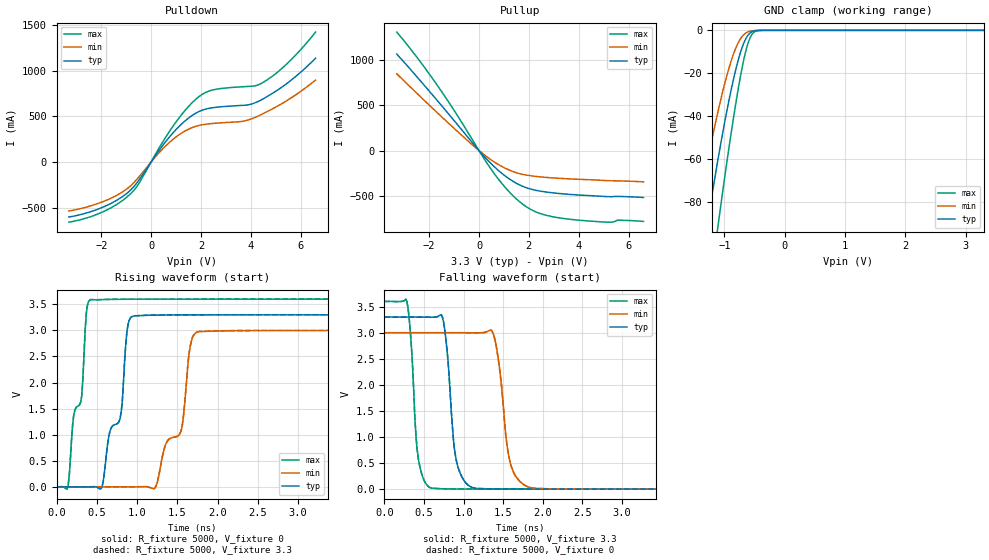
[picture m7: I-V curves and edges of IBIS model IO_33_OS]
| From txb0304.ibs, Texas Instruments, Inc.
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[Model]   IO_33_OS
Model_type  I/O
Vinl=1.05
Vinh=2.34
Enable   Active-High
Vref =   0
Rref =   5000
Cref =   15p
Vmeas =   1.65
| variable   typ   min   max
C_comp   3.56pF   3.29pF   3.85pF
| C_pullup   6.78pF   4.93pF   8.55pF
| C_pulldown   6.52pF   2.81pF   9.96pF
| C_tri-state   3.56pF   3.29pF   3.85pF
[Temperature Range]   40   100   -40
| Ambient temperature   25   85   -40
[Voltage range]   3.3   3   3.6
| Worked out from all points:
|   slope of the pulldown table from 0 to 0.495 V, typ, clamps not added: 2.58 ohm
|   slope of the pullup table from 0 to 0.495 V, typ, clamps not added: 3.39 ohm
|   GND clamp passes 1 mA (typ) near -0.56 V on its own axis
|   rising waveform, R_fixture 5000, V_fixture 0: 20-80 % time 234ps typ, 317ps min, 172ps max; typ from 0 V to 3.3 V
|   falling waveform, R_fixture 5000, V_fixture 3.3: 20-80 % time 103ps typ, 128ps min, 82.7ps max; typ from 3.3 V to 0.002 V
|   rising waveform, R_fixture 5000, V_fixture 3.3: 20-80 % time 234ps typ, 317ps min, 172ps max; typ from 0.002 V to 3.3 V
|   falling waveform, R_fixture 5000, V_fixture 0: 20-80 % time 103ps typ, 128ps min, 82.7ps max; typ from 3.3 V to 0 V
[GND Clamp]
| IO_33
|   Voltage   I(typ)   I(min)   I(max)
-3.3V     -511mA     -429.4mA   -605.2mA
-1.49V    -128.8mA   -92.59mA   -176mA
-1.305V   -94.44mA   -64.67mA   -134.3mA
-1.27V    -88.18mA   -59.68mA   -126.6mA
-1.105V   -60.01mA   -37.73mA   -91.07mA
-955mV    -36.96mA   -20.66mA   -60.66mA
-835mV    -21.06mA   -9.955mA   -38.29mA
-710mV    -8.29mA    -2.997mA   -17.96mA
-620mV    -2.726mA   -874.7uA   -7.07mA
-530mV    -508.5uA   -191.3uA   -1.442mA
-410mV    -26.79uA   -12.71uA   -53.57uA
3.3V      1.563nA    31.42nA    89.95pA
[Pulldown]
| IO_33
|   Voltage   I(typ)   I(min)   I(max)
-3.3V     -601.6mA   -536.2mA   -657.8mA
-1.9V     -489.5mA   -429.7mA   -540.3mA
-815mV    -303.8mA   -258.4mA   -344.5mA
-505mV    -203.4mA   -167.4mA   -240mA
755mV     280mA      219.3mA    342.4mA
1.365V    450.2mA    339.9mA    565.3mA
1.915V    551.4mA    399.5mA    713.7mA
2.525V    595.7mA    423.1mA    791.4mA
3.695V    620.1mA    446.7mA    823.6mA
4.46V     685.1mA    525mA      865.1mA
5.455V    860.5mA    672.7mA    1.075A
6.6V      1.135A     896.9mA    1.421A
[Pullup]
| IO_33
|   Voltage   I(typ)   I(min)   I(max)
-3.3V     1.06A      843.1mA    1.301A
-2.485V   808.2mA    627.1mA    1.022A
-1.625V   533.5mA    403.2mA    697.3mA
-850mV    280.2mA    206.8mA    377.5mA
120mV     -37.65mA   -26.89mA   -53.09mA
950mV     -257.4mA   -179.2mA   -371.9mA
1.73V     -389.7mA   -260mA     -583.6mA
2.385V    -441.5mA   -286.7mA   -684.7mA
3.28V     -472.9mA   -305.6mA   -741.3mA
5.115V    -505mA     -329.5mA   -785.6mA
5.595V    -503.5mA   -332.8mA   -764.8mA
6.6V      -515.1mA   -343.1mA   -777.6mA
[Ramp]
| IO_33
| variable   typ   min   max
dV/dt_r   2.00/2.37E-10   1.82/3.20E-10   2.19/1.73E-10
dV/dt_f   2.01/1.08E-10   1.83/1.34E-10   2.19/8.63E-11
R_load = 5000
[Rising Waveform]
| IO_33
R_fixture =   5000
C_fixture =   0
L_fixture =   0
V_fixture =   0
V_fixture_min = 0
V_fixture_max = 0
|   Time   V(typ)   V(min)   V(max)
0s        1.658nV    7.82nV     214.9pV
145ps     -6.519uV   48.58nV    31.42mV
425ps     1.627mV    -563.8nV   3.59V
789ps     1.307V     13.49uV    3.595V
901ps     3.187V     -93.83uV   3.596V
1.139ns   3.289V     -3.05mV    3.597V
1.545ns   3.296V     1.064V     3.598V
1.699ns   3.297V     2.9V       3.598V
1.993ns   3.297V     2.988V     3.598V
67.55ns   3.298V     2.997V     3.598V
[Falling Waveform]
| IO_33
R_fixture =   5000
C_fixture =   0
L_fixture =   0
V_fixture =   3.3
V_fixture_min = 3
V_fixture_max = 3.6
|   Time   V(typ)   V(min)   V(max)
0s        3.3V       3V         3.6V
285ps     3.3V       3V         3.59V
439ps     3.3V       3V         487mV
719ps     3.345V     3V         8.876mV
915ps     500.4mV    3V         3.753mV
1.265ns   9.382mV    3.006V     2.028mV
1.405ns   5.05mV     2.794V     1.824mV
1.601ns   2.935mV    436mV      1.666mV
1.937ns   1.992mV    13.15mV    1.545mV
67.55ns   1.582mV    1.775mV    1.448mV
[Rising Waveform]
| IO_33
R_fixture =   5000
C_fixture =   0
L_fixture =   0
V_fixture =   3.3
V_fixture_min = 3
V_fixture_max = 3.6
|   Time   V(typ)   V(min)   V(max)
0s        1.582mV    1.775mV    1.448mV
145ps     1.576mV    1.775mV    32.87mV
425ps     3.21mV     1.774mV    3.591V
789ps     1.309V     1.788mV    3.597V
901ps     3.19V      1.681mV    3.598V
1.139ns   3.291V     -1.276mV   3.599V
1.545ns   3.298V     1.067V     3.6V
1.699ns   3.299V     2.903V     3.6V
1.993ns   3.299V     2.991V     3.6V
67.55ns   3.3V       3V         3.6V
[Falling Waveform]
| IO_33
R_fixture =   5000
C_fixture =   0
L_fixture =   0
V_fixture =   0
V_fixture_min = 0
V_fixture_max = 0
|   Time   V(typ)   V(min)   V(max)
0s        3.298V     2.997V     3.598V
285ps     3.298V     2.997V     3.588V
439ps     3.298V     2.997V     485mV
719ps     3.343V     2.997V     7.417mV
915ps     497.8mV    2.998V     2.301mV
1.265ns   7.784mV    3.003V     579.3uV
1.405ns   3.46mV     2.791V     375.5uV
1.601ns   1.35mV     432.8mV    217.8uV
1.937ns   408.6uV    11.35mV    96.49uV
67.55ns   40.19nV    116.6nV    22.59nV
